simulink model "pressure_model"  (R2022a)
settings: Solver=VariableStepAuto  StartTime=0.0  StopTime=tfin  RelTol=1e-3
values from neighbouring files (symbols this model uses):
  Ts = 5    [sisopres.m]

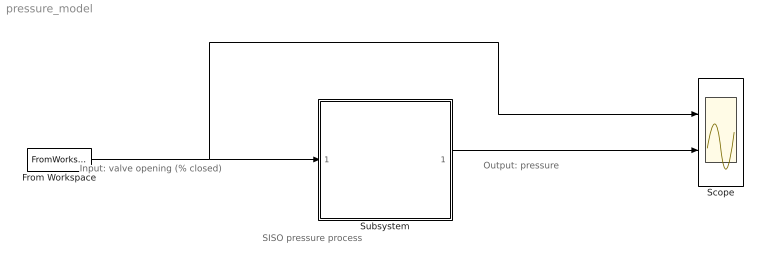
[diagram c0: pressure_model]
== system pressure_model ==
  note: Output: pressure
  note: Input: valve opening (% closed)
  note: SISO pressure process
  From Workspace : FromWorkspace  VariableName=[tsim U]  SampleTime=Ts
  Scope : Scope  NumInputPorts=2
  Subsystem : Subsystem
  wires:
  From Workspace/1 -> Scope/1, Subsystem/1(u)
  Subsystem/1(y) -> Scope/2

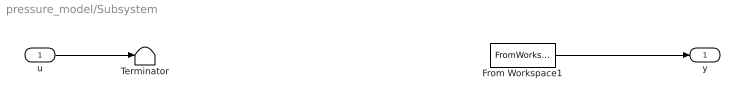
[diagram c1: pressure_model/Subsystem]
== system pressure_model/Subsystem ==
  u : Inport
  From Workspace1 : FromWorkspace  VariableName=[tsim Y]  SampleTime=Ts
  Terminator : Terminator
  y : Outport
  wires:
  From Workspace1/1 -> y/1
  u/1 -> Terminator/1
